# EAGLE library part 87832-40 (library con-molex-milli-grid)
HEADER
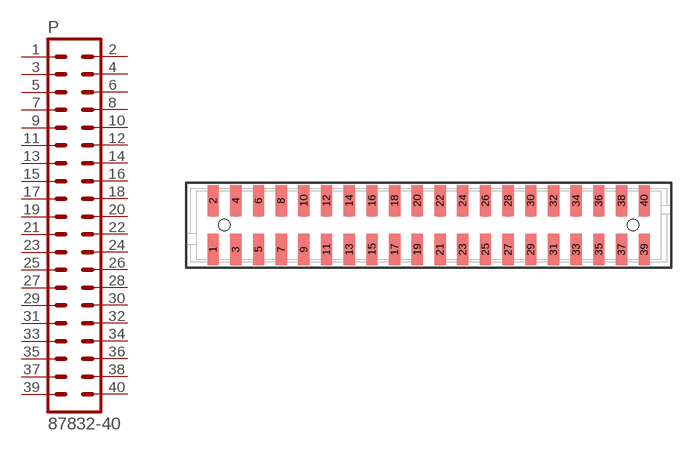
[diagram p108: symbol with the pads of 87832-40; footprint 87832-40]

Designator prefix P

## 87832-40  [87832-40]
1  1  pas
2  2  pas
3  3  pas
4  4  pas
5  5  pas
6  6  pas
7  7  pas
8  8  pas
9  9  pas
10  10  pas
11  11  pas
12  12  pas
13  13  pas
14  14  pas
15  15  pas
16  16  pas
17  17  pas
18  18  pas
19  19  pas
20  20  pas
21  21  pas
22  22  pas
23  23  pas
24  24  pas
25  25  pas
26  26  pas
27  27  pas
28  28  pas
29  29  pas
30  30  pas
31  31  pas
32  32  pas
33  33  pas
34  34  pas
35  35  pas
36  36  pas
37  37  pas
38  38  pas
39  39  pas
40  40  pas

## Footprint 87832-40 (pad centres in mm)
HEADER SMD Dual Row, Shrouded, Vertical
smd 1 x 2.75: 1 -19,-2.15; 2 -19,2.15; 3 -17,-2.15; 4 -17,2.15; 5 -15,-2.15; 6 -15,2.15; 7 -13,-2.15; 8 -13,2.15; 9 -11,-2.15; 10 -11,2.15; 11 -9,-2.15; 12 -9,2.15; 13 -7,-2.15; 14 -7,2.15; 15 -5,-2.15; 16 -5,2.15; 17 -3,-2.15; 18 -3,2.15; 19 -1,-2.15; 20 -1,2.15; 21 1,-2.15; 22 1,2.15; 23 3,-2.15; 24 3,2.15; 25 5,-2.15; 26 5,2.15; 27 7,-2.15; 28 7,2.15; 29 9,-2.15; 30 9,2.15; 31 11,-2.15; 32 11,2.15; 33 13,-2.15; 34 13,2.15; 35 15,-2.15; 36 15,2.15; 37 17,-2.15; 38 17,2.15; 39 19,-2.15; 40 19,2.15
hole 1 at -18,0
hole 1 at 18,0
